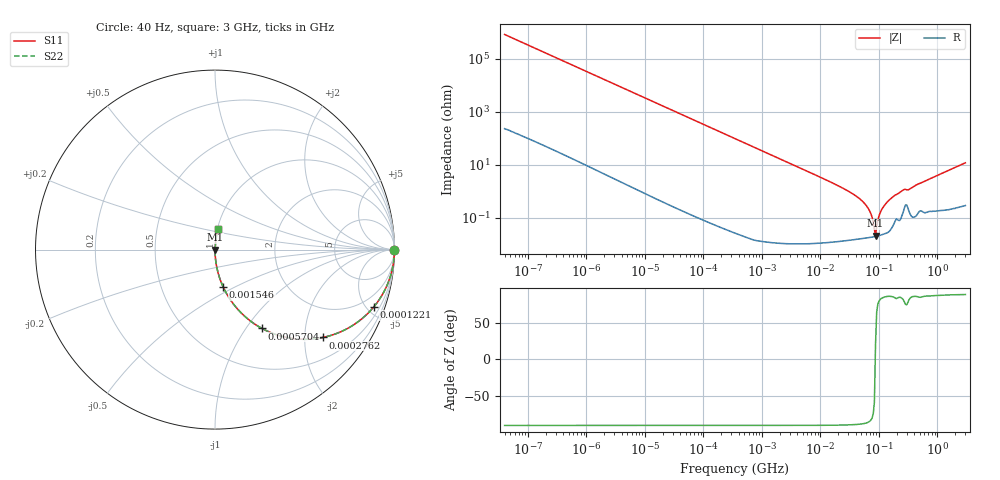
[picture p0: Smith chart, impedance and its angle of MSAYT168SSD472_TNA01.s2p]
! MSAYT168SSD472_TNA01  S-PARAMETER MODEL  ( General Type )
! Model Generated by TAIYO YUDEN Corporation (http://www.ty-top.com)
! Version 2.0
! TAIYO YUDEN Control No. 030711
! Copyright(c) 2003 TAIYO YUDEN CO.,LTD. All Rights Reserved.
! Product Description (link to TY-COMPAS)
! https://ds.yuden.co.jp/TYCOMPAS/or/detail?pn=MSAYT168SSD472KTNA01&u=M
! Products Name : Multilayer Ceramic Capacitors
! Characteristics :
!  Capacitance : 4700 pF , Rated Voltage : 25V
!  Case Size : 1.6 x 0.8 / 0.063 x 0.031 [mm/inch] , Thickness : 0.8 / 0.031 [mm/inch]
!  (Conditions: Temperature = 25 degC , DC Bias Current/Voltage = 0A / 0V)
! External Node Assignments :
!  1  o---| |---o  2
! GND o---------o GND
! Frequency Range : 40Hz  -  3GHz  [ 401 STEP ]
# MHz S RI R 50
! Freq[MHz].  S11 Real  S11 Imag  S21 Real  S21 Imag  S12 Real  S12 Imag  S22 Real  S22 Imag
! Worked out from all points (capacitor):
!   401 points, 40 Hz to 3 GHz, reference 50 ohm
!   read as one part in series: C = 4.69 nF near 44 Hz
!   lowest |Z| = 20.4 mohm at 87.39 MHz (marker M1)
!   series resonance near 86.64 MHz, so ESL is about 720 pH
!   S11 on the Smith chart (normalised r, x): 40 Hz: open; 122.1 kHz: 1.00, -5.56; 276.2 kHz: 1.00, -2.46; 570.4 kHz: 1.00, -1.19; 1.546 MHz: 1.00, -0.44; 3 GHz: 1.01, +0.24
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4e-05  1 -0.000118  4.6e-08 0.000118  4.6e-08 0.000118  1 -0.000118
0.000834  1 -0.00246  6.72e-06 0.00246  6.72e-06 0.00246  1 -0.00246
0.017386  0.9974 -0.0511  0.00263 0.0511  0.00263 0.0511  0.9974 -0.0511
0.04932  0.9793 -0.1423  0.0207 0.1423  0.0207 0.1423  0.9793 -0.1423
0.122117  0.8854 -0.3184  0.1146 0.3184  0.1146 0.3184  0.8854 -0.3184
0.276155  0.6018 -0.4894  0.3982 0.4894  0.3982 0.4894  0.6018 -0.4894
0.362475  0.4673 -0.4988  0.5327 0.4988  0.5327 0.4988  0.4673 -0.4988
0.570368  0.2617 -0.4394  0.7383 0.4394  0.7383 0.4394  0.2617 -0.4394
1.546262  0.0461 -0.2094  0.9539 0.2094  0.9539 0.2094  0.0461 -0.2094
7.222098  0.00228 -0.0466  0.9977 0.0466  0.9977 0.0466  0.00228 -0.0466
24.56009  0.000291 -0.0127  0.9997 0.0127  0.9997 0.0127  0.000291 -0.0127
46.32945  0.000183 -0.00523  0.9998 0.00523  0.9998 0.00523  0.000183 -0.00523
66.58224  0.000179 -0.00209  0.9998 0.00209  0.9998 0.00209  0.000179 -0.00209
72.90103  0.000181 -0.00137  0.9998 0.00137  0.9998 0.00137  0.000181 -0.00137
79.8195  0.000185 -0.000651  0.9998 0.000651  0.9998 0.000651  0.000185 -0.000651
87.39454  0.000191 7.34e-05  0.9998 -7.34e-05  0.9998 -7.34e-05  0.000191 7.34e-05
91.44753  0.000195 0.000417  0.9998 -0.000417  0.9998 -0.000417  0.000195 0.000417
109.6283  0.000224 0.00188  0.9998 -0.00188  0.9998 -0.00188  0.000224 0.00188
150.5692  0.000325 0.00465  0.9997 -0.00465  0.9997 -0.00465  0.000325 0.00465
259.4108  0.00171 0.0109  0.9983 -0.0109  0.9983 -0.0109  0.00171 0.0109
325.4065  0.00186 0.0114  0.9981 -0.0114  0.9981 -0.0114  0.00186 0.0114
3000  0.0166 0.1161  0.9834 -0.1161  0.9834 -0.1161  0.0166 0.1161
